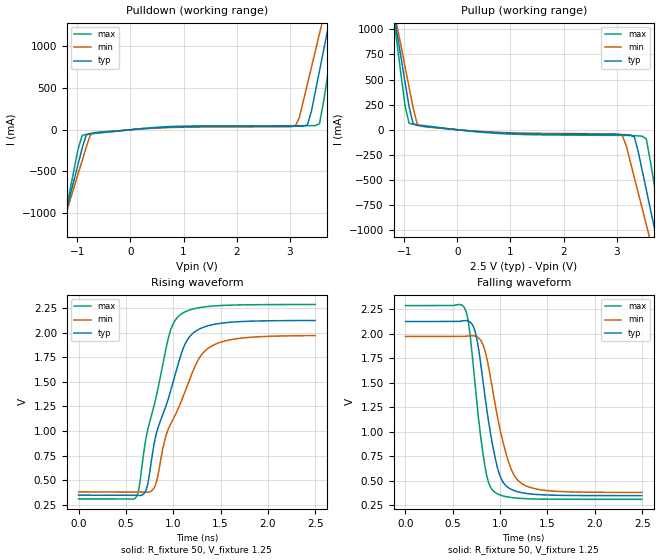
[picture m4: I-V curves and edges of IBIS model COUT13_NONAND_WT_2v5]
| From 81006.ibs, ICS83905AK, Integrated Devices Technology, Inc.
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[Model] COUT13_NONAND_WT_2v5
Model_type   Output
Polarity   Non-Inverting
|   typ   min   max
C_comp   2pF   1.5pF   2.5pF
Vmeas = 1.25V
Rref = 50
Cref = 50
Vref = 1.25V
|   typ   min   max
[Voltage range]   2.5V   2.375V   2.625V
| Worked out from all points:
|   slope of the pulldown table from 0 to 0.375 V, typ, clamps not added: 19.6 ohm
|   slope of the pullup table from 0 to 0.375 V, typ, clamps not added: 21.5 ohm
|   rising waveform, R_fixture 50, V_fixture 1.25: 20-80 % time 309ps typ, 361ps min, 257ps max; typ from 0.349 V to 2.12 V
|   falling waveform, R_fixture 50, V_fixture 1.25: 20-80 % time 170ps typ, 208ps min, 136ps max; typ from 2.12 V to 0.349 V
[Pulldown]
|Voltage   I (typ)   I (min)   I (max)
-2.5V     -4.21A     -3.7A      -5.068A
-1.364V   -1.361A    -1.321A    -1.44A
-1.288V   -1.17A     -1.162A    -1.198A
-909.1mV  -218mA     -367.5mA   -67.2mA
-833.3mV  -64.34mA   -208.7mA   -55.07mA
-681.8mV  -38.2mA    -35.6mA    -44.46mA
3.106V    41.58mA    46.68mA    48.58mA
3.333V    57.56mA    549mA      48.9mA
3.561V    704.8mA    1.153A     72.58mA
3.712V    1.188A     1.557A     639.5mA
3.864V    1.673A     1.961A     1.257A
5V        5.321A     5.003A     5.911A
[Pullup]
|Voltage   I (typ)   I (min)   I (max)
-2.5V     5.353A     4.699A     6.458A
-1.212V   1.204A     1.237A     1.169A
-1.136V   960mA      1.033A     857.5mA
-909.1mV  228.1mA    423mA      64.88mA
-681.8mV  37.67mA    34.77mA    44.41mA
3.106V    -48.31mA   -56.3mA    -56.18mA
3.333V    -71.24mA   -473.9mA   -58.81mA
3.485V    -411.7mA   -788.8mA   -64.81mA
3.561V    -600.6mA   -946.5mA   -93.28mA
3.712V    -978.7mA   -1.262A    -556.2mA
3.864V    -1.357A    -1.578A    -1.039A
5V        -4.198A    -3.948A    -4.66A
[Ramp]
|   typ   min   max
dV/dt_r   1.423/0.42n   1.273/0.496n   1.583/0.345n
dV/dt_f   1.427/0.256n   1.278/0.316n   1.589/0.201n
R_load =   50.0000
[Rising Waveform]
R_fixture = 50
V_fixture = 1.25   |Vcc_typ
V_fixture_min = 1.1875 |Vcc_min
V_fixture_max = 1.3125 |Vcc_max
C_fixture = 0.0p
| Time   typ   min   max
0s        348.7mV    381.2mV    311.1mV
613.1ps   346.7mV    381.3mV    336.1mV
718.2ps   415.8mV    377.8mV    958.7mV
803.3ps   897.3mV    433.1mV    1.282V
961ps     1.372V     1.049V     1.993V
1.069ns   1.737V     1.265V     2.178V
1.151ns   1.931V     1.47V      2.223V
1.261ns   2.03V      1.72V      2.252V
1.421ns   2.082V     1.872V     2.271V
2.498ns   2.124V     1.97V      2.286V
[Falling Waveform]
R_fixture = 50
V_fixture = 1.25   |Vcc_typ
V_fixture_min = 1.1875 |Vcc_min
V_fixture_max = 1.3125 |Vcc_max
C_fixture = 0.0p
| Time   typ   min   max
0s        2.124V     1.972V     2.286V
628.1ps   2.133V     1.973V     2.254V
675.7ps   2.122V     1.978V     2.043V
748.2ps   1.973V     1.97V      1.346V
848.3ps   1.299V     1.793V     599.9mV
938.4ps   774.3mV    1.326V     387.1mV
1.006ns   532.7mV    993.7mV    352.6mV
1.091ns   426.9mV    686.3mV    333.2mV
1.234ns   377.8mV    468.6mV    319.7mV
2.498ns   348.7mV    381.4mV    311.1mV
